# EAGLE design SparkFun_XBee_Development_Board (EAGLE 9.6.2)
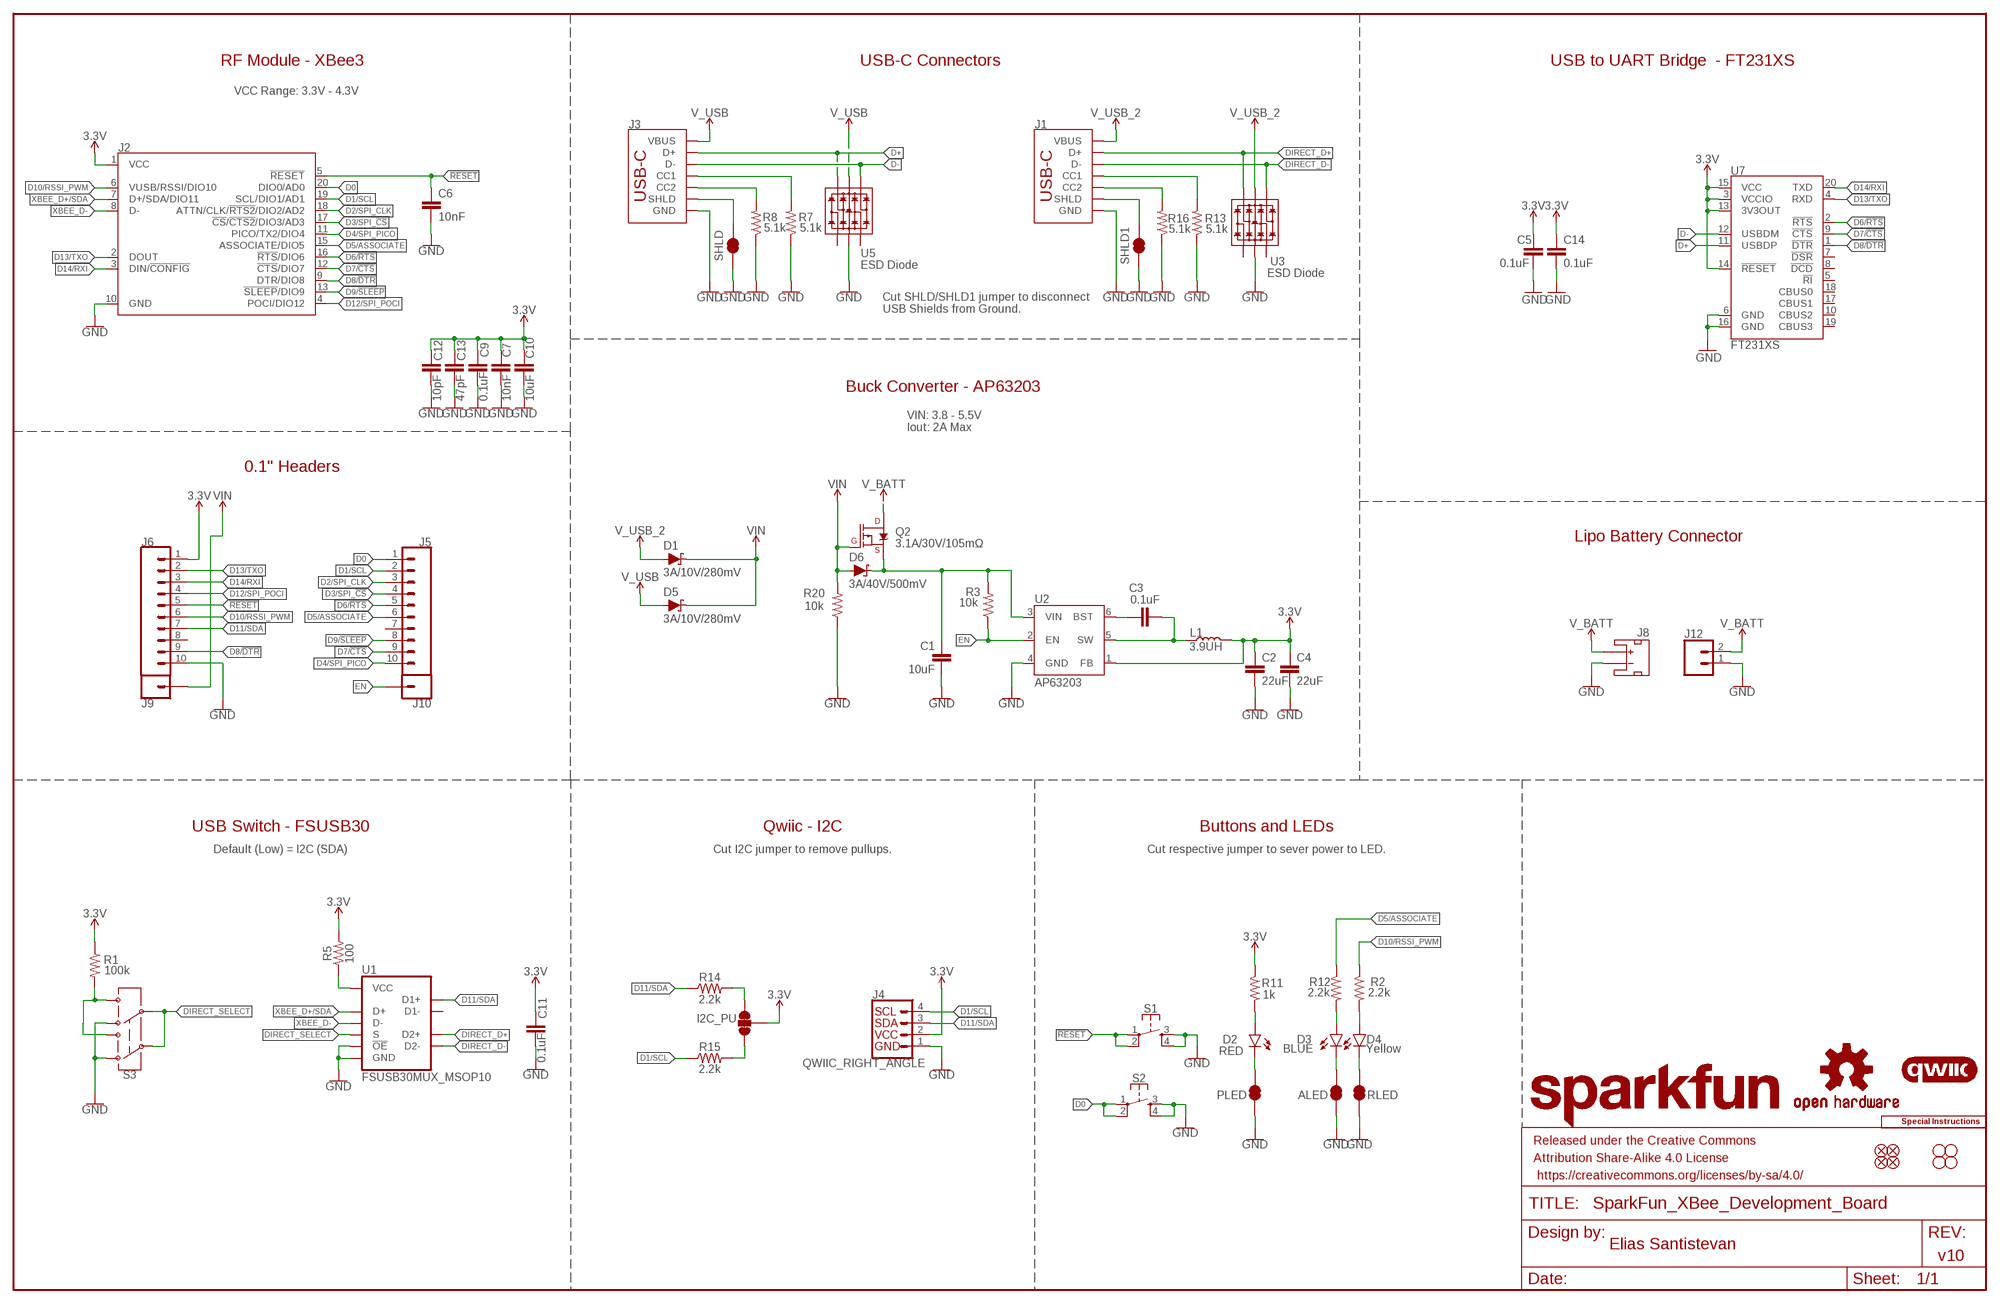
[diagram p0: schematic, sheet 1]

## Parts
ALED  JUMPER-SMT_2_NC_TRACE_SILK  [SMT-JUMPER_2_NC_TRACE_SILK]
C1  10uF  10UF-1210-50V-20%  [1210]
C2  22uF  22UF-0603-6.3V-20%  [0603]
C3  0.1uF  0.1UF-0603-25V-5%  [0603]
C4  22uF  22UF-0603-6.3V-20%  [0603]
C5  0.1uF  0.1UF-0603-25V-(+80/-20%)  [0603]
C6  10nF  10NF-0603-50V-10%  [0603]
C7  10nF  10NF-0603-50V-10%  [0603]
C9  0.1uF  0.1UF-0603-25V-(+80/-20%)  [0603]
C10  10uF  10UF-0603-6.3V-20%  [0603]
C11  0.1uF  0.1UF-0603-25V-(+80/-20%)  [0603]
C12  10pF  10PF-0603-50V-5%  [0603]
C13  47pF  47PF-0603-50V-5%  [0603]
C14  0.1uF  0.1UF-0603-25V-(+80/-20%)  [0603]
D1  3A/10V/280mV  DIODE-SCHOTTKY-BAT60A  [SOD-323]
D2  RED  LED-RED0603  [LED-0603]
D3  BLUE  LED-BLUE0603  [LED-0603]
D4  Yellow  LED-YELLOW0603  [LED-0603]
D5  3A/10V/280mV  DIODE-SCHOTTKY-BAT60A  [SOD-323]
D6  3A/40V/500mV  DIODE-SCHOTTKY-B340A  [SMA-DIODE]
FD1  FIDUCIAL1X2  [FIDUCIAL-1X2]
FD2  FIDUCIAL1X2  [FIDUCIAL-1X2]
FD3  FIDUCIAL1X2  [FIDUCIAL-1X2]
FD4  FIDUCIAL1X2  [FIDUCIAL-1X2]
FRAME1  FRAME-LEDGER  [CREATIVE_COMMONS]
H1  STAND-OFFTIGHT  [STAND-OFF-TIGHT]
H2  STAND-OFFTIGHT  [STAND-OFF-TIGHT]
H3  STAND-OFFTIGHT  [STAND-OFF-TIGHT]
H4  STAND-OFFTIGHT  [STAND-OFF-TIGHT]
I2C_PU  JUMPER-SMT_3_2-NC_TRACE_SILK  [SMT-JUMPER_3_2-NC_TRACE_SILK]
J1  USB Female Type C Connector  USB_C_4-LAYER-ISOLATED  [USB-C-16P-4LAYER-ISOLATED]
J2  XBEE_UPDATEXBEE_SMD  [XBEE3-SMD]
J3  USB Female Type C Connector  USB_C_4-LAYER-ISOLATED  [USB-C-16P-4LAYER-ISOLATED]
J4  QWIIC_RIGHT_ANGLE  QWIIC_CONNECTORJS-1MM  [JST04_1MM_RA]
J5  CONN_10NO_SILK_PTH_FEMALE  [1X10_NO_SILK]
J6  CONN_10NO_SILK_PTH_FEMALE  [1X10_NO_SILK]
J8  JST_2MM_MALE  [JST-2-SMD]
J9  CONN_01PTH_NO_SILK_STAND  [1X01_NO_SILK_STAND]
J10  CONN_01PTH_NO_SILK_STAND  [1X01_NO_SILK_STAND]
J12  CONN_021X02_NO_SILK  [1X02_NO_SILK]
L1  3.9UH  [INDUCTOR_3.9UH]
LOGO1  SFE_LOGO_NAME.2_INCH  [SFE_LOGO_NAME_.2]
LOGO2  OSHW-LOGOS  [OSHW-LOGO-S]
LOGO3  QWIIC_LOGO_5MM  [QWIIC_5MM]
LOGO5  SPECIAL_INSTRUCTIONS-ORDERING  [ORDERING_INSTRUCTIONS]
PLED  JUMPER-SMT_2_NC_TRACE_SILK  [SMT-JUMPER_2_NC_TRACE_SILK]
Q2  3.1A/30V/105mΩ  MOSFET_PCH-DMG2307L  [SOT23-3]
R1  100k  100KOHM-0603-1/10W-1%  [0603]
R2  2.2k  2.2KOHM-0603-1/10W-1%  [0603]
R3  10k  10KOHM-0603-1/10W-1%  [0603]
R5  100  100OHM-0603-1/10W-1%  [0603]
R7  5.1k  5.1KOHM5.1KOHM-0603-1/10W-1%  [0603]
R8  5.1k  5.1KOHM5.1KOHM-0603-1/10W-1%  [0603]
R11  1k  1KOHM-0603-1/10W-1%  [0603]
R12  2.2k  2.2KOHM-0603-1/10W-1%  [0603]
R13  5.1k  5.1KOHM5.1KOHM-0603-1/10W-1%  [0603]
R14  2.2k  2.2KOHM-0603-1/10W-1%  [0603]
R15  2.2k  2.2KOHM-0603-1/10W-1%  [0603]
R16  5.1k  5.1KOHM5.1KOHM-0603-1/10W-1%  [0603]
R20  10k  10KOHM-0603-1/10W-1%  [0603]
RLED  JUMPER-SMT_2_NC_TRACE_SILK  [SMT-JUMPER_2_NC_TRACE_SILK]
S1  MOMENTARY-SWITCH-SPST-2-SMD-5.2MM-TALL  [TACTILE_SWITCH_SMD_5.2MM]
S2  MOMENTARY-SWITCH-SPST-2-SMD-5.2MM-TALL  [TACTILE_SWITCH_SMD_5.2MM]
S3  SWITCH-DPDT-SMD-AYZ0202  [SWITCH_DPDT_SMD_AYZ0202]
SHLD  JUMPER-SMT_2_NC_TRACE_SILK  [SMT-JUMPER_2_NC_TRACE_SILK]
SHLD1  JUMPER-SMT_2_NC_TRACE_SILK  [SMT-JUMPER_2_NC_TRACE_SILK]
U1  FSUSB30MUX_MSOP10  [MSOP10]
U2  AP63203  [SOT23-6]
U3  ESD Diode  TVS_DIODE_ARRAY_DT1042-04SO-7  [SOT-23-6]
U5  ESD Diode  TVS_DIODE_ARRAY_DT1042-04SO-7  [SOT-23-6]
U7  FT231XS  [SSOP20_L]

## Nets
3.3V: C2.1 C4.1 C5.1 C7.1 C9.1 C10.1 C11.1 C12.1 C13.1 C14.1 I2C_PU.2 J2.1(VCC) J4.2 J6.1 L1.P$2 R1.1 R5.2 R11.1 U2.1(FB) U7.3(VCCIO) U7.13(3V3OUT) U7.14(!RESET) U7.15(VCC)
!RESET!: C6.1 J2.5(!RESET!) J6.5 S1.1 S1.2
ALED: ALED.2 D3.C
D0: J2.20(DIO0/AD0) J5.1 S2.1 S2.2
D1/SCL: J2.19(SCL/DIO1/AD1) J4.4 J5.2 R15.1
D2/SPI_CLK: J2.18(ATTN/CLK/!RTS2!/DIO2/AD2) J5.3
D3/SPI_!CS!: J2.17(!CS!/!CTS2!/DIO3/AD3) J5.4
D4/SPI_PICO: J2.11(PICO/TX2/DIO4) J5.10
D5/ASSOCIATE: J2.15(ASSOCIATE/DIO5) J5.6 R12.1
D6/!RTS!: J2.16(!RTS!/DIO6) J5.5 U7.2(!RTS)
D7/!CTS!: J2.12(!CTS!/DIO7) J5.9 U7.9(!CTS)
D8/!DTR!: J2.9(DTR/DIO8) J6.9 U7.1(!DTR)
D9/!SLEEP!: J2.13(!SLEEP!/DIO9) J5.8
D10/RSSI_PWM: J2.6(VUSB/RSSI/DIO10) J6.6 R2.1
D11/SDA: J4.3 J6.7 R14.1 U1.2(D1+)
D12/SPI_POCI: J2.4(POCI/DIO12) J6.4
D13/TXO: J2.2(DOUT) J6.2 U7.4(RXD)
D14/RXI: J2.3(DIN/!CONFIG!) J6.3 U7.20(TXD)
D+ [Diff pairs]: J3.A6(D+) J3.B6(D+) U5.6(IO4) U7.11(USBDP)
D- [Diff pairs]: J3.A7(D-) J3.B7(D-) U5.4(IO3) U7.12(USBDM)
DIRECT_D+ [Diff pairs]: J1.A6(D+) J1.B6(D+) U1.3(D2+) U3.6(IO4)
DIRECT_D- [Diff pairs]: J1.A7(D-) J1.B7(D-) U1.7(D2-) U3.4(IO3)
DIRECT_SELECT: S3.2 S3.5 U1.1(S)
EN: J10.1 R3.1 U2.2(EN)
FIRMWARE: R1.2 S3.1 S3.4
GND: ALED.1 C1.2 C2.2 C4.2 C5.2 C6.2 C7.2 C9.2 C10.2 C11.2 C12.2 C13.2 C14.2 J1.GND J1.GND2(GND) J2.10(GND) J3.GND J3.GND2(GND) J4.1 J6.10 J8.1(-) J12.1 PLED.1 R7.1 R8.1 R13.1 R16.1 R20.1 RLED.1 S1.3 S1.4 S2.3 S2.4 S3.3 S3.6 SHLD1.1 SHLD.1 U1.5(GND) U1.9(!OE!) U2.4(GND) U3.2(VSS) U5.2(VSS) U7.6(GND) U7.16(GND)
N$1: C3.1 U2.6(BST)
N$2: D4.A R2.2
N$3: R5.1 U1.10(VCC)
N$4: J3.B5(CC2) R8.2
N$5: J3.A5(CC1) R7.2
N$7: D2.A R11.2
N$8: C3.2 L1.P$1 U2.5(SW)
N$11: I2C_PU.3 R14.2
N$12: D3.A R12.2
N$13: I2C_PU.1 R15.2
N$14: J1.B5(CC2) R16.2
N$15: C1.1 D6.C Q2.2(S) R3.2 U2.3(VIN)
N$16: J1.A5(CC1) R13.2
PLED: D2.C PLED.2
RLED: D4.C RLED.2
SHLD: J3.SHLD1(SHLD) J3.SHLD2(SHLD) J3.SHLD3(SHLD) J3.SHLD4(SHLD) J3.SHLD5(SHLD) J3.SHLD6(SHLD) J3.SHLD7(SHLD) J3.SHLD8(SHLD) SHLD.2
SHLD1: J1.SHLD1(SHLD) J1.SHLD2(SHLD) J1.SHLD3(SHLD) J1.SHLD4(SHLD) J1.SHLD5(SHLD) J1.SHLD6(SHLD) J1.SHLD7(SHLD) J1.SHLD8(SHLD) SHLD1.2
V_BATT [POWER]: J8.2(+) J12.2 Q2.3(D)
V_USB: D5.A J3.VBUS1(VBUS) J3.VBUS2(VBUS) U5.5(VCC)
V_USB_2: D1.A J1.VBUS1(VBUS) J1.VBUS2(VBUS) U3.5(VCC)
VIN: D1.C D5.C D6.A J9.1 Q2.1(G) R20.2
XBEE_D+/SDA [Diff pairs]: J2.7(D+/SDA/DIO11) U1.4(D+)
XBEE_D- [Diff pairs]: J2.8(D-) U1.6(D-)
Unconnected: J5.7 J6.8 J8.NC1(PAD1) J8.NC2(PAD2) U1.8(D1-) U3.1(IO1) U3.3(IO2) U5.1(IO1) U5.3(IO2) U7.5(!RI) U7.7(!DSR) U7.8(!DCD) U7.10(CBUS2) U7.17(CBUS1) U7.18(CBUS0) U7.19(CBUS3)

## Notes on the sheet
- RF Module - XBee3 | USB-C Connectors | USB to UART Bridge  - FT231XS
- VCC Range: 3.3V - 4.3V
- Cut SHLD/SHLD1 jumper to disconnect
  USB Shields from Ground.
- Buck Converter - AP63203
- VIN: 3.8 - 5.5V
  Iout: 2A Max
- 0.1" Headers
- Lipo Battery Connector
- USB Switch - FSUSB30 | Qwiic - I2C | Buttons and LEDs
- Default (Low) = I2C (SDA) | Cut I2C jumper to remove pullups. | Cut respective jumper to sever power to LED.
- Elias Santistevan
- v10

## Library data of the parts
ALED PLED RLED SHLD SHLD1 = SparkFun-Jumpers:JUMPER-SMT_2_NC_TRACE: Normally closed trace jumper
C1 = SparkFun-Capacitors:10UF: 10.0µF ceramic capacitors; PROD_ID: CAP-09824
C2 C4 = SparkFun-Capacitors:22UF: 22µF ceramic capacitors; PROD_ID: CAP-14464
C3 = SparkFun-Capacitors:0.1UF: 0.1µF ceramic capacitors; PROD_ID: CAP-08604
C5 C9 C11 C14 = SparkFun-Capacitors:0.1UF: 0.1µF ceramic capacitors; PROD_ID: CAP-00810
C6 C7 = SparkFun-Capacitors:10NF: 0.01uF/10nF/10,000pF ceramic capacitors; PROD_ID: CAP-00867
C10 = SparkFun-Capacitors:10UF: 10.0µF ceramic capacitors; PROD_ID: CAP-11015
C12 = SparkFun-Capacitors:10PF: 10pF ceramic capacitors; PROD_ID: CAP-11812
C13 = SparkFun-Capacitors:47PF: 47pF ceramic capacitors; PROD_ID: CAP-08913
D1 D5 = SparkFun-DiscreteSemi:DIODE-SCHOTTKY: Schottky diode; PROD_ID: DIO-14072
D2 = SparkFun-LED:LED-RED: Red SMD LED; PROD_ID: DIO-00819
D3 = SparkFun-LED:LED-BLUE: Blue SMD LED; PROD_ID: DIO-08575
D4 = SparkFun-LED:LED-YELLOW: Yellow SMD LED; PROD_ID: DIO-09003
D6 = SparkFun-DiscreteSemi:DIODE-SCHOTTKY: Schottky diode; PROD_ID: DIO-09886
FD1-FD4 = SparkFun-Aesthetics:FIDUCIAL: Fiducial Alignment Points
FRAME1 = SparkFun-Aesthetics:FRAME-LEDGER: Schematic Frame - Ledger
H1-H4 = SparkFun-Hardware:STAND-OFF: Stand Off
I2C_PU = SparkFun-Jumpers:JUMPER-SMT_3_2-NC_TRACE: Normally closed trace jumper (2 of 2 connections) This jumper has a trace between all three pads so they are normally closed (NC). Use a razor knife to open the connection(s). For best results follow the IPC guidelines for cutting traces: Cutout at least 0.063 mm (0.005 in). Remove all loose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
J1 J3 = SparkFun-Connectors:USB_C: USB Type C 16Pin Connector Super Speed pins not available on the 16-pin purely SMD connector so this part is best for USB 2.0 implementations. D1 and D2 are tied together enabling D+/- no matter which way the cable is plugged into the connector. The two channel configuration pins (CC1/2) are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; PROD_ID: CONN-14122
J2 = xbee_smart_modem:XBEE_UPDATE: XBee 3 Cat 1 Smart Modem
J4 = SparkFun-Connectors:QWIIC_CONNECTOR: SparkFun I2C Standard Qwiic Connector An SMD 1mm pitch JST connector makes it easy and quick (get it? Qwiic?) to connect I2C devices to each other. The Qwiic system enables fast and solderless connection between popular platforms and various sensors and actuators. We carry 200mm, 100mm, 50mm, and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; PROD_ID: CONN-13694
J5 J6 = SparkFun-Connectors:CONN_10: Multi connection point. Often used as Generic Header-pin footprint for 0.1 inch spaced/style header connections On any of the 0.1 inch spaced packages, you can populate with these: Break Away Headers - Straight (PRT-00116) Break Away Male Headers - Right Angle (PRT-00553) Female Headers (PRT-00115)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
J8 = SparkFun-Connectors:JST_2MM_MALE: JST 2MM MALE RA CONNECTOR Two pin, compact surface mount connector. Commonly used as a battery input connection point. We really like the solid locking feeling and high current rating on these small connectors. We use these all the time as battery connectors. Mates to single-cell LiPo batteries.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; PROD_ID: CONN-11443; SF_ID: PRT-08612
J9 J10 = SparkFun-Connectors:CONN_01: Single connection point. Often used as Generic Header-pin footprint for 0.1 inch spaced/style header connections
J12 = SparkFun-Connectors:CONN_02: Multi connection point. Often used as Generic Header-pin footprint for 0.1 inch spaced/style header connections
L1 = SparkFun-Coils:3.9UH: Würth's Electronik 3.9uH Inductor
LOGO1 = SparkFun-Aesthetics:SFE_LOGO_NAME: SparkFun Font Logo
LOGO2 = SparkFun-Aesthetics:OSHW-LOGO: Open-Source Hardware (OSHW) Logo
LOGO3 = SparkFun-Aesthetics:QWIIC_LOGO: Qwiic Logos for placement on schematic and PCB. The 5.5mm silk logo is best for placing next to Qwiic connector.
LOGO5 = SparkFun-Aesthetics:SPECIAL_INSTRUCTIONS: Special Ordering/Production Instructions Alert
Q2 = SparkFun-DiscreteSemi:MOSFET_PCH: P-channel MOSFETs Voltage controlled devices that allow control of high current outputs. SparkFun Products: SparkFun ESP32 Thing SparkFun ESP8266 Thing SparkFun Pi Servo HAT V2 DMG2305UX-7 (20V/4.2A/SOT23-3); PROD_ID: TRANS-11308
R1 = SparkFun-Resistors:100KOHM: 100kΩ resistor; PROD_ID: RES-07828
R2 R12 R14 R15 = SparkFun-Resistors:2.2KOHM: 2.2kΩ resistor; PROD_ID: RES-08272
R3 R20 = SparkFun-Resistors:10KOHM: 10kΩ resistor; PROD_ID: RES-00824
R5 = SparkFun-Resistors:100OHM: 100Ω resistor; PROD_ID: RES-07863
R7 R8 R13 R16 = SparkFun-Resistors:5.1KOHM; PROD_ID: RES-12083
R11 = SparkFun-Resistors:1KOHM: 1kΩ resistor; PROD_ID: RES-07856
S1 S2 = SparkFun-Switches:MOMENTARY-SWITCH-SPST-2: Momentary Switch (Pushbutton) - SPST - Two Circuits Normally-open (NO) SPST momentary switches (buttons, pushbuttons). Schematic symbol includes two switch circuits. Variants SMD-4.6MMX2.8MM - 4.60mm x 2.80mm Tactile Momentary Button Switch - Used on SparkFun Pro Micro - RP2040 SMD-5.2MM - Mini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; PROD_ID: SWCH-14139
S3 = SparkFun-Switches:SWITCH-DPDT: Double-Pole, Double-Throw (DPDT) Switch Double-pole, double-throw switches. Variant Overview PTH-GPI-152-3013 Used on SparkFun Geiger Counter SMD-AY0202 Surface Mount DPDT Switch (COM-00597) Used on e.g. LilyPad Arduino USB - ATmega32U4 Board; PROD_ID: SWCH-08179; SF_SKU: COM-00597
U1 = SparkFun-IC-Special-Function:FSUSB30MUX; PROD_ID: IC-15569
U2 = SparkFun-IC-Power:AP63203: Diodes Inc. AP63203 3.8V-32V input 3.3V Buck The AP63200/AP63201/AP63203/AP63205 is a 2A, synchronous buck converter with a wide input voltage range of 3.8V to 32V and fully integrates a 125mΩ high-side power MOSFET and a 68mΩ lowside power MOSFET to provide high-efficiency step-down DC/DC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; PROD_ID: VREG-15244
U3 U5 = SparkFun-DiscreteSemi:TVS_DIODE_ARRAY; PROD_ID: IC-13538
U7 = SparkFun-IC-Comms:FT231X: FTDI FT231X Full Speed USB to Full-handshake UART This USB2.0 Full Speed IC offers a compact bridge to full handshake UART interfaces. The device is a UART, capable of operating up to 3MBaud, with low power consumption (8mA). The FT231X includes the complete FT-X series feature set and enables USB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; PROD_ID: IC-11524

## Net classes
1 POWER: width 0.559 mm, drill 0.305 mm
2 Diff pairs: width 0.203 mm, drill 0.305 mm, clearance 0.152 mm

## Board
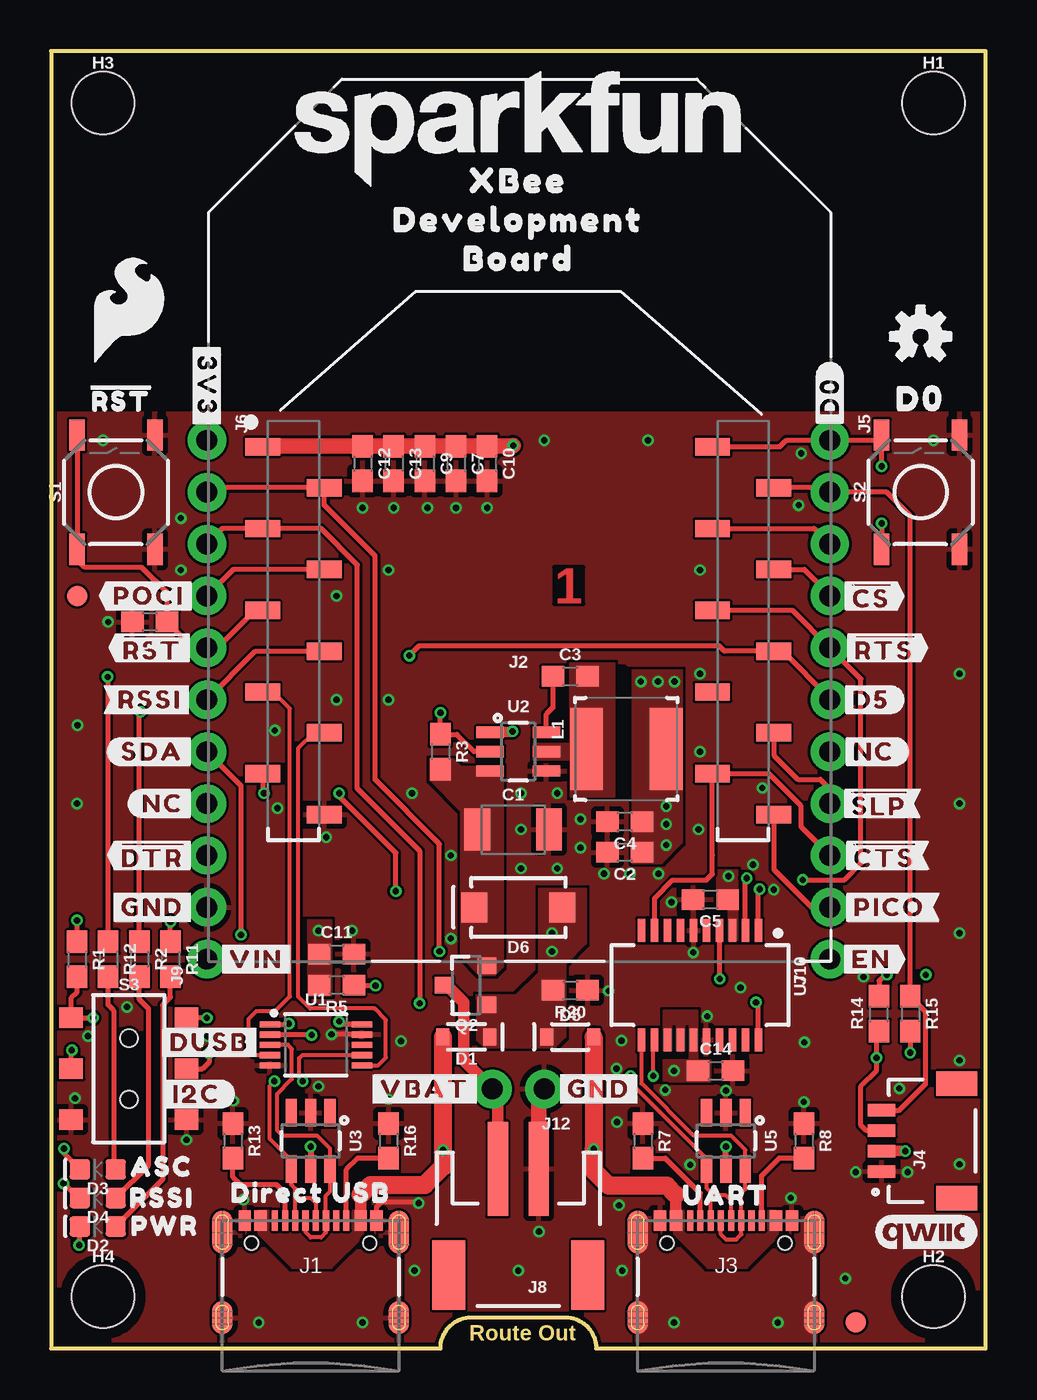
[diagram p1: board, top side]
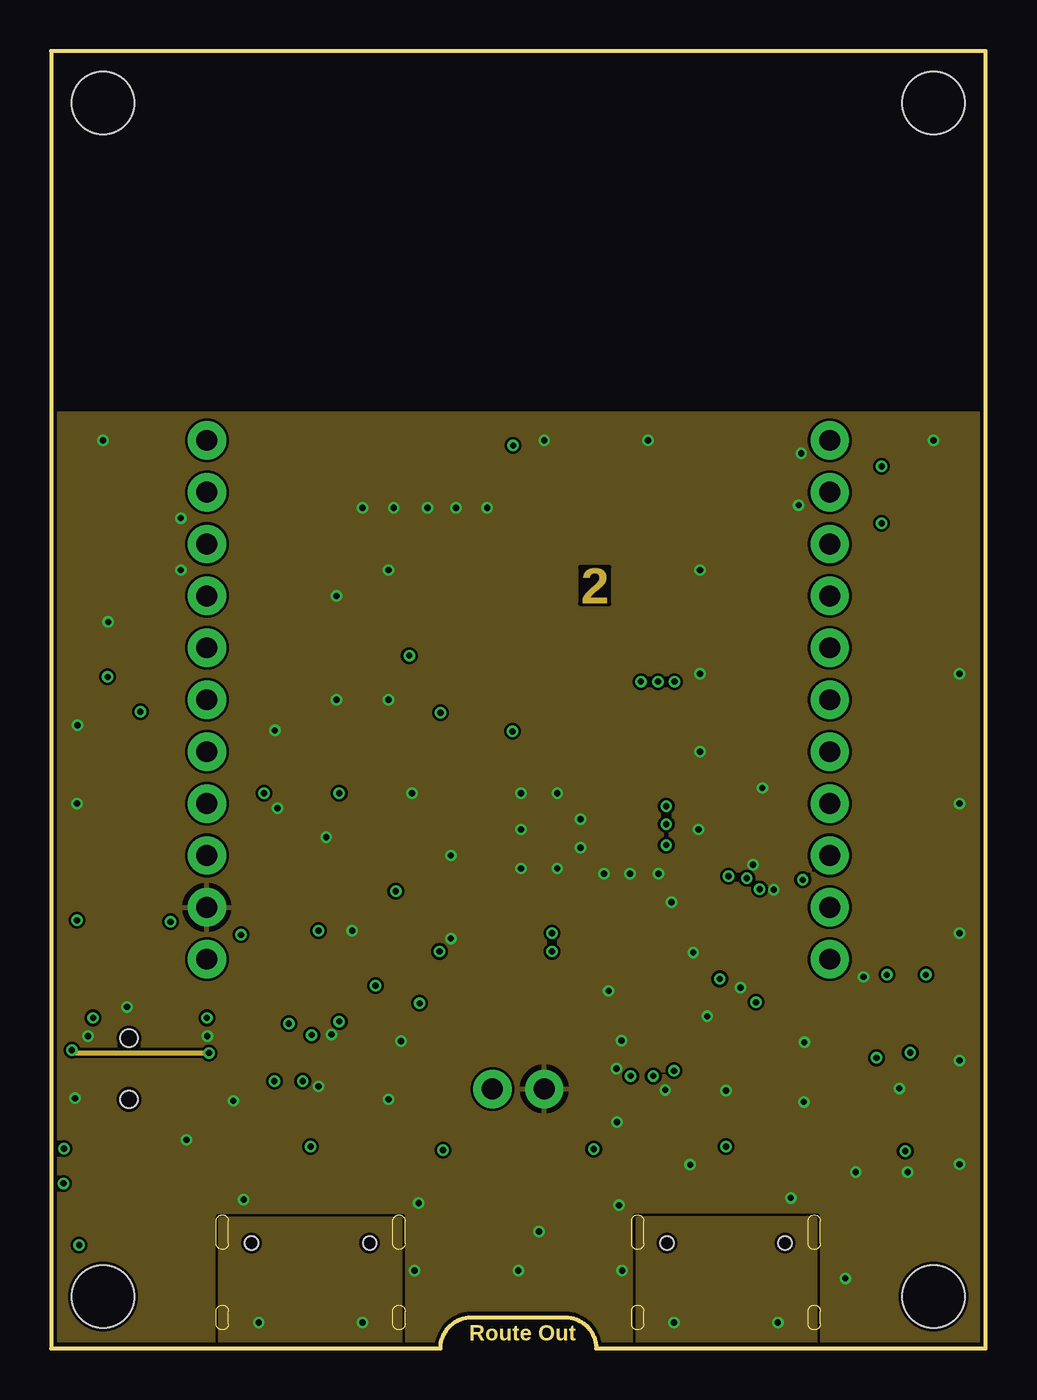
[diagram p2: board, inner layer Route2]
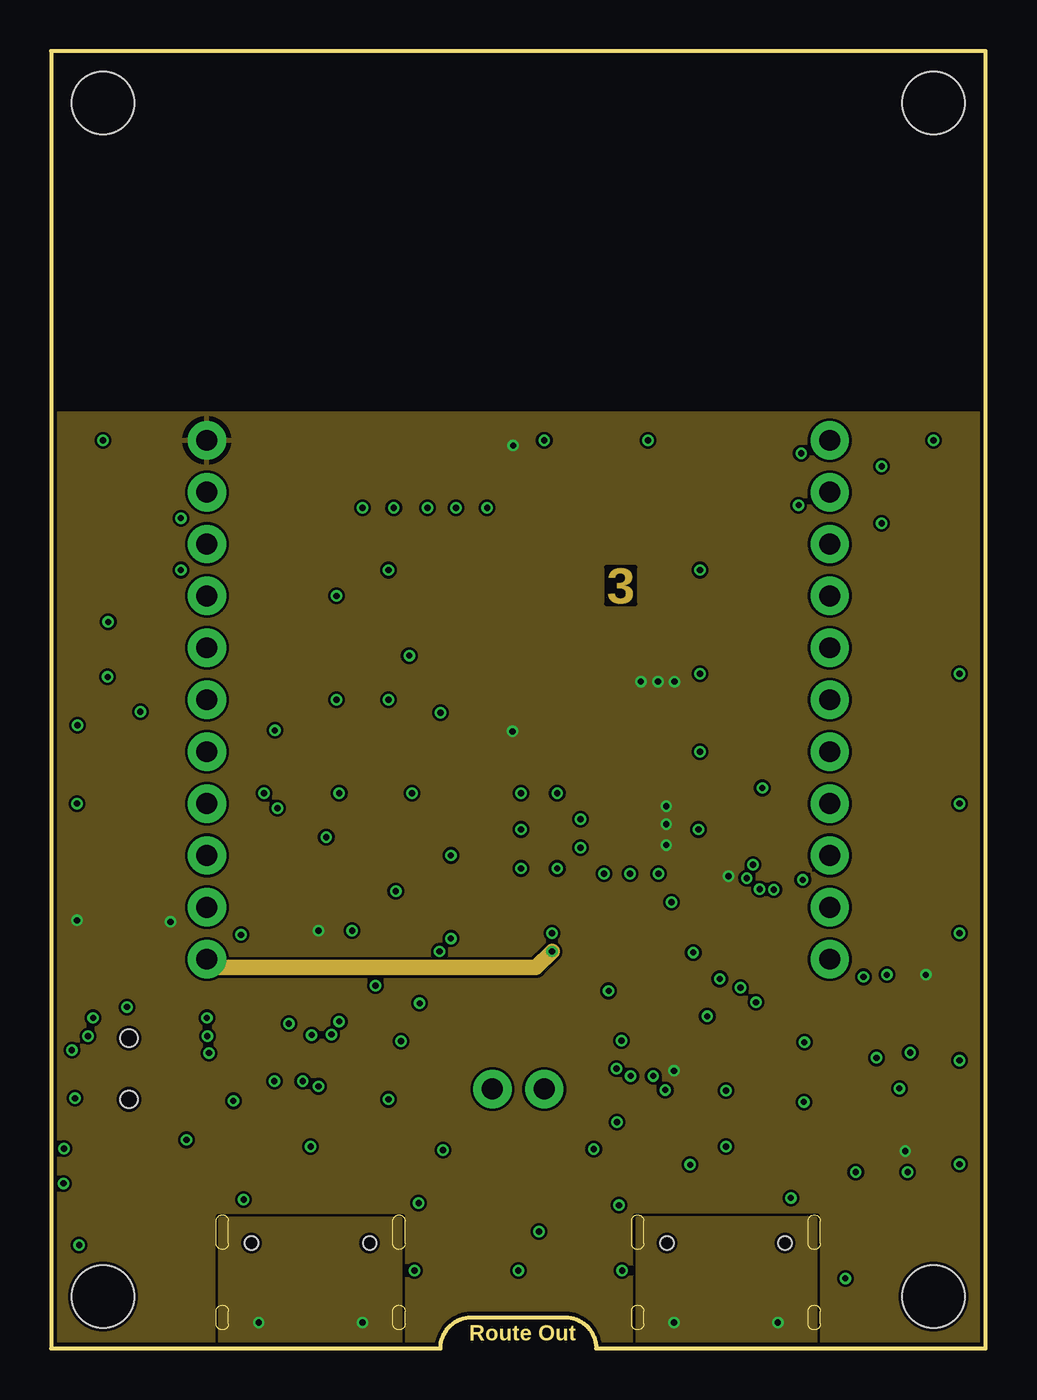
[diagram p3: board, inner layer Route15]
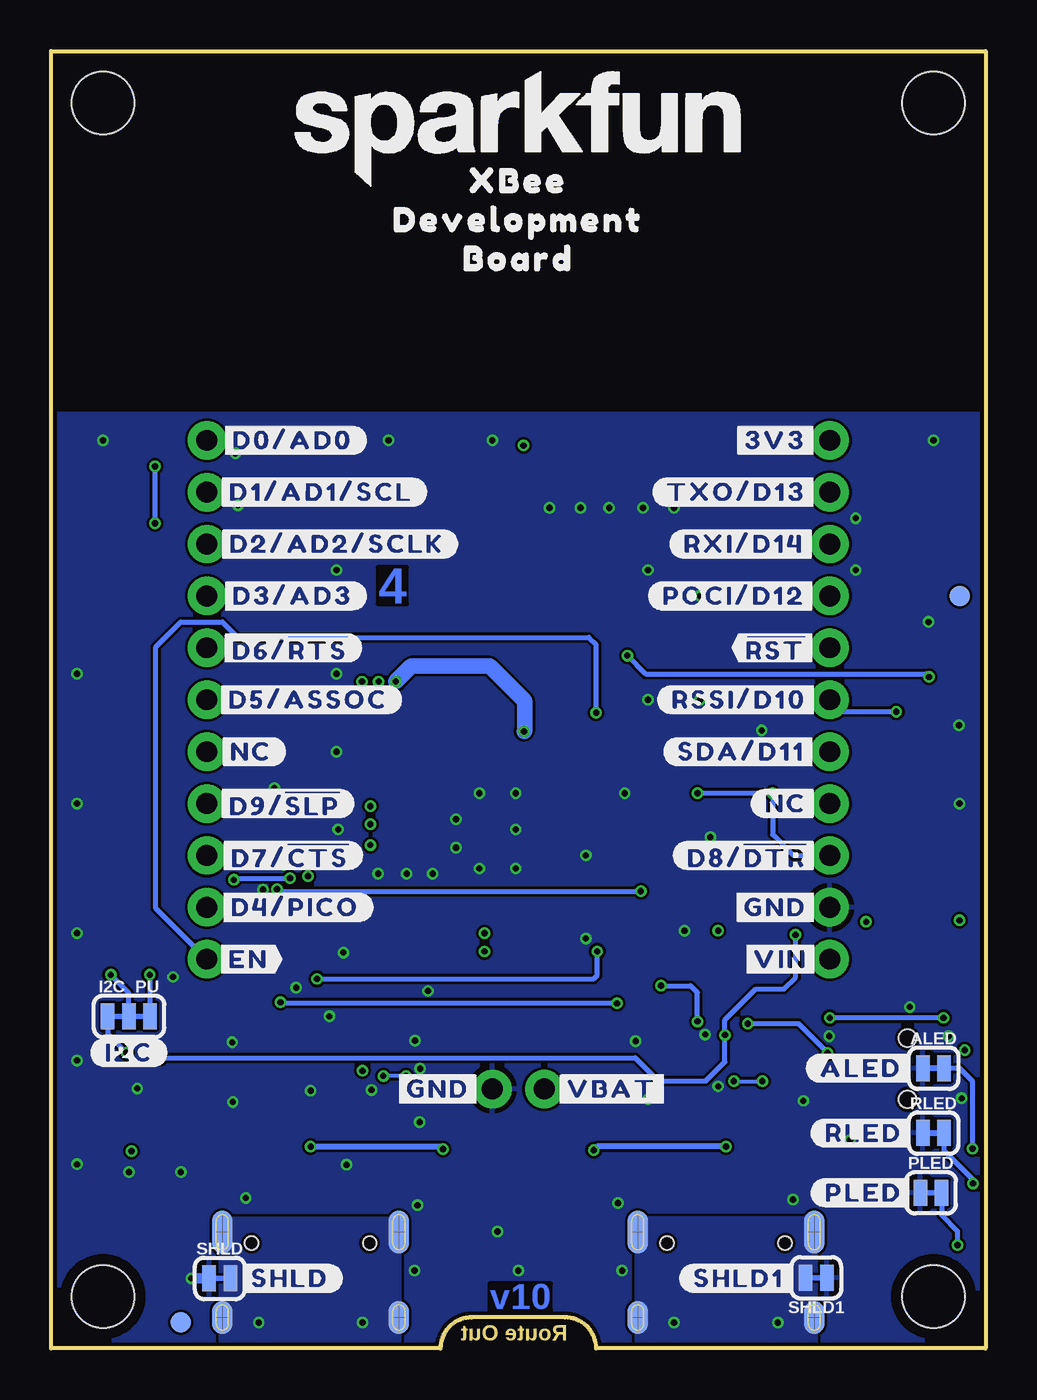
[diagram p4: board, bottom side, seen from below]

Size 45.72 x 63.5 mm. Coordinates in mm from the lower left corner, seen from the top.
Outline: 0,63.5 0,0 19.05,0 arc-90 20.57,1.52 25.15,1.52 arc-90 26.67,0 45.72,0 45.72,63.5 0,63.5
Copper layers (1*2*15*16): Top 0.035559375mm / dielectric 0.47751875mm / Route2 0.035559375mm / dielectric 0.47751875mm / Route15 0.035559375mm / dielectric 0.47751875mm / Bottom 0.035559375mm
Design rules "SparkFun-4-Layer-Minimum-JLCPCB": minimum track width 5mil, minimum drill 0.2mm, track to track 5mil, track to pad 5mil, pad to pad 5mil, via to via 5mil, smd to smd 5mil, copper to edge 7mil, drill to drill 7mil, minimum pad ring 5mil, minimum via ring 5mil, stop-mask expansion 2.5mil, vias tented up to drill 25mil, thermal gap 10mil
tRestrict: area 27.8,33.1 to 28.1,33.4; area 27.9,26.9 to 28.1,27.2

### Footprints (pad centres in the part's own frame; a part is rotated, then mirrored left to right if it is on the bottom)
SMT-JUMPER_2_NC_TRACE_SILK = smd 0.66 x 1.27: 1 -0.521,0; 2 0.521,0
1210 = smd 1.27 x 2.06: 1 -1.755,0; 2 1.755,0
0603 = smd 1.1 x 1: 1 -0.85,0; 2 0.85,0
SOD-323 = smd 0.63 x 0.83: A 1.15,0; C -1.15,0
LED-0603 = smd 1 x 1: A -0.877,0; C 0.877,0
SMA-DIODE = smd 1.27 x 1.47: A -2.15,0; C 2.15,0
FIDUCIAL-1X2 = smd 1 x 1: 1 0,0
STAND-OFF-TIGHT = hole 3.048: 0,0
SMT-JUMPER_3_2-NC_TRACE_SILK = smd 0.66 x 1.27: 1 -1.041,0; 2 0,0; 3 1.041,0
USB-C-16P-4LAYER-ISOLATED = smd 0.3 x 1: A5 -1.25,-0.34; A6 -0.25,-0.34; A7 0.25,-0.34; A8 1.25,-0.34; B5 1.75,-0.34; B6 0.75,-0.34; B7 -0.75,-0.34; B8 -1.75,-0.34 | smd 0.6 x 1: GND -3.225,-0.34; GND2 3.225,-0.34; VBUS1 -2.45,-0.34; VBUS2 2.45,-0.34 | smd 1 x 2.1: SHLD1 -4.32,-0.915; SHLD2 4.32,-0.915 | smd 1 x 2.1 bottom: SHLD3 -4.32,-0.915; SHLD4 4.32,-0.915 | smd 1 x 1.6: SHLD5 -4.32,-5.095; SHLD8 4.32,-5.095 | smd 1 x 1.6 bottom: SHLD6 -4.32,-5.095; SHLD7 4.32,-5.095 | hole 0.65: -2.89,-1.445; 2.89,-1.445
XBEE3-SMD = smd 1.7 x 0.85: 1 -12.5,11.11; 2 -9.5,9.11; 3 -12.5,7.11; 4 -9.5,5.11; 5 -12.5,3.11; 6 -9.5,1.11; 7 -12.5,-0.89; 8 -9.5,-2.89; 9 -12.5,-4.89; 10 -9.5,-6.89; 11 12.5,-6.89; 12 9.5,-4.89; 13 12.5,-2.89; 14 9.5,-0.89; 15 12.5,1.11; 16 9.5,3.11; 17 12.5,5.11; 18 9.5,7.11; 19 12.5,9.11; 20 9.5,11.11
JST04_1MM_RA = smd 0.6 x 1.35: 1 -1.5,0; 2 -0.5,0; 3 0.5,0; 4 1.5,0 | smd 1.2 x 2: NC1 2.8,-3.675; NC2 -2.8,-3.675
1X10_NO_SILK = drill 1.016 pad 1.88: 1 0,0; 2 2.54,0; 3 5.08,0; 4 7.62,0; 5 10.16,0; 6 12.7,0; 7 15.24,0; 8 17.78,0; 9 20.32,0; 10 22.86,0
JST-2-SMD = smd 1 x 4.6: 1 -1,-3.7; 2 1,-3.7 | smd 1.6 x 3.4: NC1 -3.4,1.5; NC2 3.4,1.5
1X01_NO_SILK_STAND = drill 1.016 pad 1.88: 1 0,0
1X02_NO_SILK = drill 1.016 pad 1.88: 1 0,0; 2 2.54,0
INDUCTOR_3.9UH = smd 4 x 1.6: P$1 0,-2; P$2 0,1.9
SOT23-3 = smd 0.8 x 0.9: 1 -0.95,-1; 2 0.95,-1; 3 0,1.1
TACTILE_SWITCH_SMD_5.2MM = smd 1.524 x 0.762: 1 -2.794,1.905; 2 2.794,1.905; 3 -2.794,-1.905; 4 2.794,-1.905
SWITCH_DPDT_SMD_AYZ0202 = smd 1 x 1.15: 1 -2.5,2.825; 2 0,2.825; 3 2.5,2.825; 4 -2.5,-2.825; 5 0,-2.825; 6 2.5,-2.825 | hole 0.85: 1.5,0; -1.5,0
MSOP10 = smd 1 x 0.3: 1 -2.25,1; 2 -2.25,0.5; 3 -2.25,0; 4 -2.25,-0.5; 5 -2.25,-1; 6 2.25,-1; 7 2.25,-0.5; 8 2.25,0; 9 2.25,0.5; 10 2.25,1
SOT23-6 = smd 0.55 x 1.35: 1 -0.95,-1.375; 2 0,-1.375; 3 0.95,-1.375; 4 0.95,1.375; 5 0,1.375; 6 -0.95,1.375
SOT-23-6 = smd 0.55 x 1.35: 1 -0.95,-1.375; 2 0,-1.375; 3 0.95,-1.375; 4 0.95,1.375; 5 0,1.375; 6 -0.95,1.375
SSOP20_L = smd 0.381 x 1.143: 1 -2.857,-2.68; 2 -2.223,-2.68; 3 -1.587,-2.68; 4 -0.953,-2.68; 5 -0.318,-2.68; 6 0.318,-2.68; 7 0.953,-2.68; 8 1.587,-2.68; 9 2.223,-2.68; 10 2.857,-2.68; 11 2.857,2.68; 12 2.223,2.68; 13 1.587,2.68; 14 0.953,2.68; 15 0.318,2.68; 16 -0.318,2.68; 17 -0.953,2.68; 18 -1.587,2.68; 19 -2.223,2.68; 20 -2.857,2.68

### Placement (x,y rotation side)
ALED  2.54,13.72 0 bottom
C1  22.61,25.4 0 top
C2  28.07,24.28 180 top
C3  25.4,32.89 0 top
C4  28.07,25.78 180 top
C5  32.26,21.97 180 top
C6  4.83,35.56 180 top
C7  19.81,43.31 270 top
C9  18.29,43.31 270 top
C10  21.34,43.31 270 top
C11  13.97,19.3 0 top
C12  15.24,43.31 270 top
C13  16.76,43.31 270 top
C14  32.51,13.59 0 top
D1  20.32,15.24 180 top
D2  2.29,5.97 180 top
D3  2.29,8.76 180 top
D4  2.29,7.37 180 top
D5  25.4,15.24 0 top
D6  22.86,21.59 180 top
FD1  1.27,36.83 0 top
FD2  1.27,36.83 0 bottom
FD3  39.37,1.27 0 top
FD4  39.37,1.27 0 bottom
FRAME1  not placed on the board
H1  43.18,60.96 0 top
H2  43.18,2.54 0 top
H3  2.54,60.96 0 top
H4  2.54,2.54 0 top
I2C_PU  41.91,16.26 0 bottom
J1  12.7,6.6 0 top
J2  22.86,33.02 0 top
J3  33.02,6.6 0 top
J4  40.64,10.16 90 top
J5  38.1,44.45 270 top
J6  7.62,44.45 270 top
J8  22.86,5.08 180 top
J9  7.62,19.05 90 top
J10  38.1,19.05 90 top
J12  24.13,12.7 180 top
L1  28.19,29.34 270 top
LOGO1  22.86,59.69 0 top
LOGO2  42.55,49.53 0 top
LOGO3  42.8,5.71 0 top
LOGO5  not placed on the board
PLED  2.67,7.62 0 bottom
Q2  20.32,17.78 90 top
R1  1.27,19.05 270 top
R2  4.32,19.05 270 top
R3  19.05,29.21 270 top
R5  13.97,17.78 180 top
R7  28.96,10.16 270 top
R8  36.83,10.16 270 top
R11  5.84,19.05 270 top
R12  2.79,19.05 270 top
R13  8.89,10.16 270 top
R14  40.51,16.38 90 top
R15  42.04,16.38 270 top
R16  16.51,10.16 270 top
R20  25.4,17.53 180 top
RLED  2.54,10.54 0 bottom
S1  3.17,41.91 90 top
S2  42.55,41.91 90 top
S3  3.81,13.69 270 top
SHLD  37.47,3.43 0 bottom
SHLD1  8.28,3.45 180 bottom
U1  12.95,14.86 0 top
U2  22.86,29.21 270 top
U3  12.7,10.16 180 top
U5  33.02,10.16 180 top
U7  31.75,17.78 180 top
U$1  [#D2#AD2#SCLK#19]  31.75,39.37 0 bottom
U$2  [##RST##15]  4.95,34.29 0 top
U$3  [##CS##19]  40.13,36.83 0 top
U$4  [##CTS##25]  40.77,24.13 0 top
U$5  [##DTR##27]  4.95,24.13 0 top
U$6  [#D1#AD1#SCL#8]  32.51,41.91 0 bottom
U$7  [##RTS##24]  40.77,34.29 0 top
U$8  [#EN#17]  40.13,19.05 0 top
U$9  [#3V3#1]  7.62,47.12 270 top
U$10  [#D0#18]  38.1,46.61 90 top
U$11  [#VBAT#5]  18.29,12.7 0 top
U$12  [#D3#AD3#22]  33.91,36.83 0 bottom
U$13  [#D4#PICO#24]  33.78,21.59 0 bottom
U$14  [#POCI#D12#24]  12.32,36.83 0 bottom
U$15  [#TXO#D13#13]  12.19,41.91 0 bottom
U$16  [#RXI#D14#15]  11.81,39.37 0 bottom
U$17  [##RST##15]  10.29,34.29 0 bottom
U$18  [#RSSI#D10#17]  12.06,31.75 0 bottom
U$20  [#GND#0]  26.8,12.7 0 top
U$21  [#EN#17]  36.07,19.05 0 bottom
U$22  [#SDA#D11#8]  11.94,29.21 0 bottom
U$23  [XBEE339]  22.86,57.15 0 top
U$24  [#NC#1]  35.94,29.21 0 bottom
U$25  [#GND#0]  4.95,21.59 0 top
U$26  [#I2C#33]  41.91,14.48 0 bottom
U$27  [#ALED#21]  6.1,13.72 0 bottom
U$28  [#PICO#23]  41.02,21.59 0 top
U$29  [#POCI#23]  4.78,36.83 0 top
U$30  [#RST#30]  3.43,46.48 0 top
U$31  [#RSSI#16]  4.83,31.75 0 top
U$32  [#DUSB#31]  7.75,14.99 0 top
U$34  [#SDA#7]  4.95,29.21 0 top
U$35  [#SHLD#30]  34.04,3.43 0 bottom
U$36  [#SHLD1#31]  12.06,3.43 0 bottom
U$37  [#VBAT#5]  18.29,12.7 0 bottom
U$38  [#GND#0]  26.8,12.7 0 bottom
U$39  [#D5#3]  40.13,31.75 0 top
U$40  [D03]  42.55,46.48 0 top
U$41  [#VIN#4]  10.03,19.05 0 top
U$42  [PWR26]  5.56,5.99 0 top
U$43  [ASC32]  5.41,8.89 0 top
U$44  [#3V3#1]  10.29,44.45 0 bottom
U$45  [#GND#0]  10.29,21.59 0 bottom
U$46  [#VIN#4]  10.03,19.05 0 bottom
U$47  [##SLP##27]  40.51,26.67 0 top
U$48  [#NC#3]  9.78,26.67 0 bottom
U$49  [#I2C#31]  7.11,12.45 0 top
U$50  [XBEE339]  22.86,57.15 0 bottom
U$51  [DEVELOPMENT1345]  22.86,55.24 0 top
U$52  [BOARD1346]  22.86,53.34 0 top
U$53  [#D8##DTR##27]  11.68,24.13 0 bottom
U$54  [#PLED#20]  5.97,7.62 0 bottom
U$55  [#D0#AD0#18]  33.91,44.45 0 bottom
U$56  [#D5#ASSOC#24]  33.15,31.75 0 bottom
U$57  [#D6##RTS##24]  34.04,34.29 0 bottom
U$58  [#D7##CTS##25]  34.04,24.13 0 bottom
U$60  [#D9##SLP##27]  34.29,26.67 0 bottom
U$61  [SFE_LOGO_FLAME_.2]  3.81,50.8 0 top
U$62  [RSSI31]  5.41,7.37 0 top
U$63  [SFE_LOGO_NAME_.2]  22.86,59.69 0 bottom
U$64  [#RLED#22]  5.97,10.54 0 bottom
U$65  [UART32]  33.02,7.49 0 top
U$66  [#NC#3]  5.46,26.67 0 top
U$67  [#NC#1]  40.26,29.21 0 top
U$68  [DIRECT_USB33]  12.7,7.62 0 top
U$70  [DEVELOPMENT1345]  22.86,55.24 0 bottom
U$71  [BOARD1346]  22.86,53.34 0 bottom

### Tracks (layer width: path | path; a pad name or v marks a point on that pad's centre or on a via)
3.3V  (via drill 0.3)
  Top 0.254: R11.1 v5.84,20.88 | R1.1 v1.27,20.95
  Top 0.508: J4.2 v41.79,9.66 | U2.1 22.54,30.16 v22.58,30.2
  Top 0.762: J2.1 10.39,44.16 C12.1 C13.1 C9.1 C7.1 C10.1 22.57,44.16 v22.61,44.2
  Bottom 0.254: I2C_PU.2 41.91,17.4 v42.8,18.29
  Bottom 0.762: v22.58,30.2 22.55,30.23 22.55,31.7 24.26,33.4 28.09,33.4 v28.85,32.64
  other vias: 30.1,25.65 30.1,26.54 30.1,24.64 29.69,32.64 30.51,32.64 30.48,13.59 33.15,23.11 13.08,20.45
  pour Top (no thermals): 28.45,23.77 28.45,33.17 30.86,33.17 30.86,24.77 29.87,23.77
  pour Route15 (isolate 0.127, rank 3): 0,0 45.72,0 45.72,45.72 0,45.72
  pour Top (no thermals): 30.48,13.08 32.26,13.08 32.26,14.1 31.62,14.1 31.62,15.62 31.62,16.51 29.97,16.51 29.97,14.61 30.35,14.61 30.35,15.88 30.61,15.88 30.61,15.75 30.61,14.61 30.99,14.61 30.99,15.88 31.24,15.88 31.24,14.61 31.24,14.1 29.97,14.1 29.97,13.08
  pour Top (no thermals): 33.15,19.99 33.15,21.51 32.59,21.51 32.59,23.39 33.07,23.39 33.58,23.39 33.58,19.99
  pour Top (no thermals): 12.57,20.95 12.57,17.27 13.72,17.27 13.72,20.95
!RESET!
  Top 0.254: J2.5 10.36,36.07 9.91,36.07 8.13,34.29 J6.5 6.95,34.29 C6.1 5.68,37 4.45,38.23 1.65,38.23 1.27,38.61 S1.1 S1.2
ALED  (via drill 0.3)
  Top 0.254: D3.C 0.64,9.54 v0.64,9.78
  Bottom 0.254: v0.64,9.78 0.64,13.08 1.27,13.72 ALED.2
D0  (via drill 0.3)
  Top 0.254: J2.20 35.66,44.13 35.98,44.45 J5.1 40.64,44.45 | v40.64,43.18 40.64,44.45 | 40.64,44.45 S2.2 | v40.64,40.39 S2.1
  Bottom 0.254: v40.64,43.18 v40.64,40.39
D1/SCL
  Top 0.254: J2.19 37.88,42.13 J5.2 40.89,41.91 42.04,40.77 R15.1 42.79,16.48 42.79,12.95 41.51,11.66 J4.4
D2/SPI_CLK
  Top 0.254: J5.3 37.34,40.13 J2.18
D3/SPI_!CS!
  Top 0.254: J2.17 36.86,38.13 38.1,36.89 J5.4
D4/SPI_PICO
  Top 0.254: J2.11 35.36,23.44 37.21,21.59 J5.10
D5/ASSOCIATE  (via drill 0.3)
  Top 0.254: v17.53,33.91 18,34.38 32.69,34.38 32.95,34.13 J2.15 35.79,34.13 38.1,31.82 J5.6 | v2.77,32.87 2.77,19.93 R12.1
  Bottom 0.254: v2.77,32.87 2.92,33.02 16.64,33.02 v17.53,33.91
D6/!RTS!  (via drill 0.3)
  Top 0.254: J2.16 36.26,36.13 J5.5 39.62,32.77 39.62,23.74 38.82,22.94 v36.78,22.94 | U7.2 33.97,22.95 v34.04,23.01
  Bottom 0.254: v36.78,22.94 36.7,23.01 v34.04,23.01
D7/!CTS!
  Top 0.254: J5.9 36.7,25.53 36.7,26.54 35.12,28.13 J2.12 32.36,24.13 32.36,23.22 32.07,22.92 30.42,22.92 29.53,22.04 U7.9
D8/!DTR!  (via drill 0.3)
  Top 0.254: v16.87,22.38 16.87,24.26 14.1,27.03 v14.1,27.18 | v10.41,27.18 10.36,27.23 J2.9 | U7.1 34.61,22.42 v34.67,22.48
  Bottom 0.254: v14.1,27.18 v10.41,27.18 10.41,25.15 9.4,24.13 J6.9 | v34.67,22.48 34.57,22.38 v16.87,22.38
D9/!SLEEP!
  Top 0.254: J5.8 38.1,27.39 37.63,27.86 36.53,27.86 35.36,29.03 J2.13
D10/RSSI_PWM  (via drill 0.3)
  Top 0.254: J6.6 10,34.13 J2.6 | v4.37,31.17 4.28,31.08 4.28,19.94 R2.1
  Bottom 0.254: J6.6 7.04,31.17 v4.37,31.17
D11/SDA  (via drill 0.3)
  Top 0.254: U1.2 12.73,15.36 v12.75,15.34 | v9.3,20.24 9.3,27.53 J6.7 | J4.3 39.89,10.66 39.62,10.92 39.62,12.83 40.39,13.59 v40.39,14.22 40.39,15.41 R14.1
  Bottom 0.254: v9.3,20.24 9.3,18.16 9.87,17.59 11.24,17.59 12.75,16.08 v12.75,15.34 12.75,14.02 13.68,13.09 16.02,13.09 17.14,14.22 v40.39,14.22
D12/SPI_POCI
  Top 0.254: J2.4 8.92,38.13 J6.4
D13/TXO  (via drill 0.3)
  Top 0.254: v19,19.43 19,24.69 15.85,27.84 15.85,38.78 13.36,41.27 J2.2 7.84,42.13 J6.2 | U7.4 32.7,18.1 v32.72,18.09
  Bottom 0.254: v19,19.43 19,18.26 19.18,18.09 v32.72,18.09
D14/RXI  (via drill 0.3)
  Top 0.254: v18.03,16.89 18.03,24.36 14.99,27.41 14.99,38.35 13.21,40.13 J2.3 8.38,40.13 J6.3 | U7.20 34.61,16.83 v34.49,16.94
  Bottom 0.254: v34.49,16.94 34.49,16.92 18.06,16.92 v18.03,16.89
D+
  Top 0.203: J3.A6 32.77,5.58 33.02,5.33 33.53,5.33 33.77,5.58 J3.B6 33.77,7.61 33.97,7.81 U5.6 33.97,9.72 33.27,10.41 31.45,10.41 28.89,12.97 U7.11
D-  (via drill 0.3)
  Top 0.203: J3.B7 32.27,7.49 | 32.27,7.49 32.27,7.64 32.07,7.84 U5.4 32.05,8.81 32.05,9.31 28.36,13 v28.36,13.34 | J3.A7 33.27,7.24 33.02,7.49 32.27,7.49 | v29.46,13.34 29.46,15.04 U7.12
  Bottom 0.203: v28.36,13.34 v29.46,13.34
DIRECT_D+
  Top 0.203: J1.A6 12.45,5.69 12.7,5.44 13.21,5.44 13.45,5.68 J1.B6 13.45,7.48 13.65,7.68 U3.6 13.65,9.78 13.02,10.41 11.33,10.41 11.05,10.69 11.05,12.45 11.79,13.18 11.79,14.66 11.58,14.86 U1.3
DIRECT_D-  (via drill 0.3)
  Top 0.203: U1.7 12.3,14.36 12.14,14.2 12.14,13.25 v12.31,13.08 | J1.B7 11.95,7.37 | 11.95,7.37 11.95,7.82 11.75,8.02 U3.4 11.75,9.21 10.69,10.27 10.69,12.85 v10.92,13.08 | 11.95,7.37 12.7,7.37 12.95,7.12 J1.A7
  Bottom 0.203: v12.31,13.08 v10.92,13.08
DIRECT_SELECT  (via drill 0.3)
  Top 0.254: v11.63,15.9 11.63,15.86 U1.1 | v1.02,14.61 0.98,14.57 S3.5 | S3.2 7.42,13.69 7.73,14 v7.73,14.46
  Route2 0.254: v1.02,14.61 1.08,14.61 1.22,14.46 v7.73,14.46
  Bottom 0.254: v11.63,15.9 9.17,15.9 v7.73,14.46
EN  (via drill 0.3)
  Top 0.254: U2.2 20.7,29.21 19.85,30.06 R3.1 v19.05,31.11
  Bottom 0.254: J10.1 40.59,21.54 40.59,34.34 39.37,35.56 37.34,35.56 36.58,34.8 19.41,34.8 19.05,34.44 v19.05,31.11
FIRMWARE  (via drill 0.3)
  Top 0.254: R1.2 1.27,17.44 0.98,17.15 S3.4 2.05,16.19 v2.06,16.18 | v7.62,16.18 v7.61,16.19 S3.1
  Bottom 0.254: v2.06,16.18 v7.62,16.18
GND  (via drill 0.3)
  Top 0.254: U1.9 v13.72,15.36 v13.72,15.37 | J1.GND2 15.93,6.92 16.15,7.14 17.95,7.14 v17.98,7.11
  Top 0.762: J8.1 23.86,12.43 J12.1
  Bottom 0.508: v38.86,3.43 SHLD.1
  other vias: 19.56,24.13 36.83,12.06 15.24,41.15 8.92,12.12 25.91,25.91 25.91,24.51 41.91,8.64 39.37,8.64 16.51,12.19 19.56,20.07 17.65,27.18 34.34,23.67 16.76,41.15 18.41,41.15 23.88,5.71 39.75,18.19 36.7,43.81 44.45,33.02 44.45,26.67 44.45,20.32 44.45,14.1 22.86,3.81 27.94,3.81 1.27,26.67 36.58,41.27 13.46,25.02 29.72,23.24 31.67,25.4 34.8,27.43 2.54,44.45 6.63,10.21 1.17,12.24 1.8,15.29 7.65,15.29 44.45,9.02 1.3,30.51 29.21,44.45 24.13,44.45 3.71,16.71 41.5,12.73 43.18,44.45 17.78,3.81 19.81,41.15 21.34,41.15 16.51,38.1 16.51,31.75 31.75,38.1 31.75,33.02 31.75,29.21 13.97,31.75 13.97,36.83 24.77,27.18 24.77,23.5 27.05,23.24 22.99,25.4 22.99,27.18 22.99,23.5 28.32,23.24 6.35,38.1 6.35,40.64 30.35,21.84 27.28,17.5 31.42,19.38 32.11,16.26 33.73,17.65 35.36,22.45 14.73,20.45 13.08,12.83 33.02,12.62 27.69,11.07 31.27,8.99 36.2,7.37 27.79,7.01 9.42,7.29 36.86,14.99 17.12,15.04 27.91,15.06 27.66,13.69 30.05,12.65 11.07,26.44 2.79,35.56 10.95,30.25
  pour Top (isolate 0.127, rank 3): 0,0 45.72,0 45.72,45.72 0,45.72
  pour Route2 (isolate 0.127, rank 3): 0,0 45.72,0 45.72,45.72 0,45.72
  pour Bottom (isolate 0.127, rank 3): 0,0 45.72,0 45.72,45.72 0,45.72
N$1
  Top 0.254: C3.1 24.55,31.36 24.23,31.05 U2.6
N$2
  Top 0.254: R2.2 4.32,17.08 4.77,16.62 4.77,8.97 D4.A
N$3  (via drill 0.3)
  Top 0.254: U1.10 14.24,15.86 v14.1,16 | v15.88,17.75 15.85,17.78 R5.1
  Bottom 0.254: v14.1,16 14.1,17.42 14.43,17.75 v15.88,17.75
N$4
  Top 0.254: J3.B5 34.77,8.46 35.62,9.31 R8.2
N$5
  Top 0.254: J3.A5 31.77,7.6 30.06,9.31 R7.2
N$7
  Top 0.254: R11.2 5.84,17.18 5.46,16.8 5.46,8.27 D2.A
N$8
  pour Top (no thermals): 23.62,28.83 25.43,28.83 25.43,27.03 27.56,27.03 27.56,33.53 25.4,33.53 25.4,29.59 23.62,29.59
N$11  (via drill 0.3)
  Top 0.254: v40.89,18.29 40.81,18.29 40.51,18 R14.2
  Bottom 0.254: I2C_PU.3 40.87,18.26 v40.89,18.29
N$12
  Top 0.254: R12.2 2.79,16.8 3.06,16.54 3.06,8.87 D3.A
N$13  (via drill 0.3)
  Top 0.254: R15.2 v42.04,14.48
  Bottom 0.254: I2C_PU.1 42.95,15.39 v42.04,14.48
N$14
  Top 0.254: J1.B5 14.45,8.76 15,9.31 R16.2
N$15
  pour Top (no thermals): 18.54,28.83 19.68,28.83 20.07,28.45 22.1,28.45 22.1,18.67 21.72,18.29 20.95,18.29 20.07,19.18 20.07,26.29 18.54,27.81
N$16
  Top 0.254: J1.A5 11.45,7.6 11.05,8 9.27,8 8.89,8.38 R13.2
PLED  (via drill 0.3)
  Top 0.254: D2.C 1.37,5.93 v1.37,5.05
  Bottom 0.254: PLED.2 2.15,6.51 1.37,5.74 v1.37,5.05
RLED  (via drill 0.3)
  Top 0.254: D4.C 1.32,7.37 v0.61,8.08
  Bottom 0.254: v0.61,8.08 0.61,8.25 2.02,9.66 RLED.2
SHLD  (via drill 0.3)
  other vias: 30.48,1.27 35.56,1.27
  pour Top (rank 2, no thermals): 28.68,6.35 28.68,0 37.39,0 37.39,6.35
  pour Bottom (rank 2, no thermals): 28.7,6.35 28.7,0 37.39,0 37.39,6.35
  pour Route2 (rank 2, no thermals): 28.7,6.35 28.7,0 37.39,0 37.39,6.35
  pour Route15 (rank 2, no thermals): 28.7,6.35 28.7,0 37.39,0 37.39,6.35
SHLD1  (via drill 0.3)
  other vias: 10.16,1.27 15.24,1.27
  pour Top (rank 2): 8.31,6.35 8.31,0 17.07,0 17.07,6.35
  pour Bottom (rank 2, no thermals): 17.07,6.35 17.07,0 8.31,0 8.31,6.35
  pour Route15 (rank 2): 17.07,6.35 17.07,0 8.31,0 8.31,6.35
  pour Route2 (rank 2): 17.07,6.35 17.07,0 8.31,0 8.31,6.35
V_BATT
  Top 0.559: J8.2 21.86,12.43 J12.2 20.19,14.1 20.19,16.93 19.35,17.78 Q2.3
V_USB  (via drill 0.3)
  Top 0.305: U5.5 v33.02,9.88
  Top 0.559: J3.VBUS1 30.57,7.53
  Top 0.889: 30.57,7.53 30.12,7.98 27.27,7.98 26.55,8.69 v26.55,9.75 D5.A
  Bottom 0.305: v33.02,9.88 26.68,9.88 v26.55,9.75
  pour Top (no thermals): 30.48,6.73 30.48,5.59 32.13,3.94 34.04,3.94 35.56,5.46 35.56,6.6 35.43,6.73
V_USB_2  (via drill 0.3)
  Top 0.305: v12.7,9.88 U3.5
  Top 0.559: J1.VBUS2 15.15,7.53
  Top 0.889: 15.15,7.53 15.62,8 18.29,8 19.17,8.88 v19.17,9.7 D1.A
  Bottom 0.305: v12.7,9.88 18.99,9.88 v19.17,9.7
  pour Top (no thermals): 10.16,6.73 10.16,5.59 11.81,3.94 13.72,3.94 15.24,5.46 15.24,6.6 15.11,6.73
VIN  (via drill 0.3)
  Route15 0.762: J9.1 8.03,18.64 23.72,18.64 v24.51,19.43
  other vias: 24.51,20.32
  pour Top (isolate 0.305, no thermals): 21.21,14.73 24.64,14.73 25.15,15.24 25.15,18.8 26.16,19.81 26.16,22.48 23.88,22.48 23.88,18.41 22.73,17.27 20.83,17.27 20.83,15.11
XBEE_D+/SDA
  Top 0.203: J2.7 11.05,32.13 11.05,31.95 11.68,31.32 11.68,17.22 10.97,16.51 10.06,16.51 9.65,16.1 9.65,14.61 9.9,14.36 U1.4
XBEE_D-
  Top 0.203: U1.6 16.02,13.86 16.38,14.22 16.38,16.08 15.82,16.64 12.68,16.64 12.1,17.21 12.1,29.38 12.85,30.13 J2.8

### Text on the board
Top: 1
Route2: 2
Route15: 3
Bottom: 4 | v10
Milling: Route Out
Measures: Units in Inches
tDocu: FOUR LAYER BOARD | 1.6mm Thickness | LEAD-FREE HASL | Elias Santistevan

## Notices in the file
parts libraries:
SparkFun-Capacitors: Licensing: Creative Commons ShareAlike 4.0 International - https://creativecommons.org/licenses/by-sa/4.0
SparkFun-Aesthetics: Released under the Creative Commons Attribution Share-Alike 4.0 License
SparkFun-Aesthetics: https://creativecommons.org/licenses/by-sa/4.0
